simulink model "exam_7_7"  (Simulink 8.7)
settings: Solver=VariableStepAuto  StartTime=0.0  StopTime=10.0  RelTol=1e-3

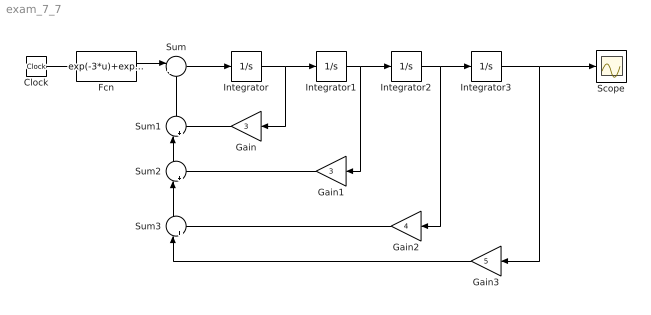
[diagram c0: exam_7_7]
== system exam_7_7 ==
  Clock : Clock
  Fcn : Fcn  Expr=exp(-3*u)+exp(-5*u)*sin(4*u+pi/3)
  Gain : Gain  Gain=3
  Gain1 : Gain  Gain=3
  Gain2 : Gain  Gain=4
  Gain3 : Gain  Gain=5
  Integrator{,1..3} (4 alike) : Integrator
  Scope : Scope
  Sum : Sum  Inputs=|+-
  Sum1 : Sum  Inputs=|++
  Sum2 : Sum  Inputs=|++
  Sum3 : Sum  Inputs=|++
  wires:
  Clock/1 -> Fcn/1
  Fcn/1 -> Sum/1
  Sum/1 -> Integrator/1
  Integrator/1 -> Gain/1, Integrator1/1
  Integrator1/1 -> Gain1/1, Integrator2/1
  Integrator2/1 -> Gain2/1, Integrator3/1
  Integrator3/1 -> Gain3/1, Scope/1
  Gain/1 -> Sum1/2
  Gain2/1 -> Sum3/2
  Gain3/1 -> Sum3/1
  Sum1/1 -> Sum/2
  Sum2/1 -> Sum1/1
  Sum3/1 -> Sum2/1
  Gain1/1 -> Sum2/2
